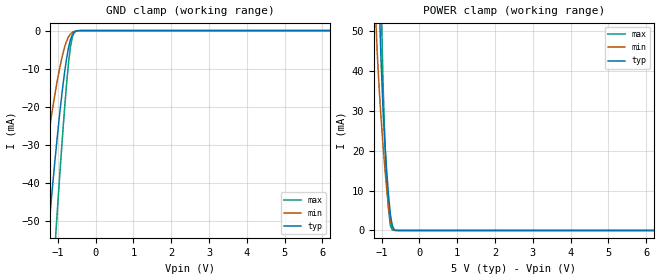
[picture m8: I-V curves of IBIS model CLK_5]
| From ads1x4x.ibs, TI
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|   CLK 5.0V Model
[Model]   CLK_5
Model_type   Input
| Signals   CLK
Vinl = 0.75V
Vinh = 2.00V
| variable   typ   min   max
C_comp   6.286pF   6.918pF   5.639pF
[Temperature Range]   40.0   105.0   -40.0
[Voltage range]   5.0V   4.75V   5.25V
[power clamp reference] 5.0V   4.75V   5.25V
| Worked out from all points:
|   GND clamp passes 1 mA (typ) near -0.61 V on its own axis
|   POWER clamp passes 1 mA (typ) near -0.71 V on its own axis
[GND Clamp]
|   Voltage   I(typ)   I(min)   I(max)
-5V       -567.3mA   -418.3mA   -701.2mA
-1.567V   -91.45mA   -52mA      -136mA
-1.266V   -54.97mA   -28.96mA   -86.89mA
-1.216V   -49.27mA   -25.52mA   -78.87mA
-1.067V   -33.09mA   -16.08mA   -55.32mA
-1.016V   -28.06mA   -13.25mA   -47.73mA
-866.5mV  -14.46mA   -6.044mA   -26.34mA
-716.5mV  -4.454mA   -1.617mA   -8.394mA
-666.5mV  -2.392mA   -893.2uA   -4.245mA
-616.5mV  -1.071mA   -469.8uA   -1.676mA
-566.5mV  -392.3uA   -240.1uA   -507.9uA
9.983V    0A         0A         0A
[POWER Clamp]
|   Voltage   I(typ)   I(min)   I(max)
-5V       2.152A     1.797A     2.717A
-1.167V   98.52mA    56.14mA    143.3mA
-1.117V   77.62mA    44.9mA     113.8mA
-1.067V   58.93mA    35.98mA    85.75mA
-1.016V   43.41mA    28.56mA    60.11mA
-966.5mV  31.54mA    21.98mA    38.61mA
-916.5mV  22.52mA    15.96mA    23.08mA
-866.5mV  15.12mA    10.52mA    12.71mA
-816.5mV  8.846mA    5.906mA    5.347mA
-766.5mV  3.971mA    2.572mA    1.183mA
-716.5mV  1.159mA    818.8uA    131.3uA
9.983V    0A         0A         0A
